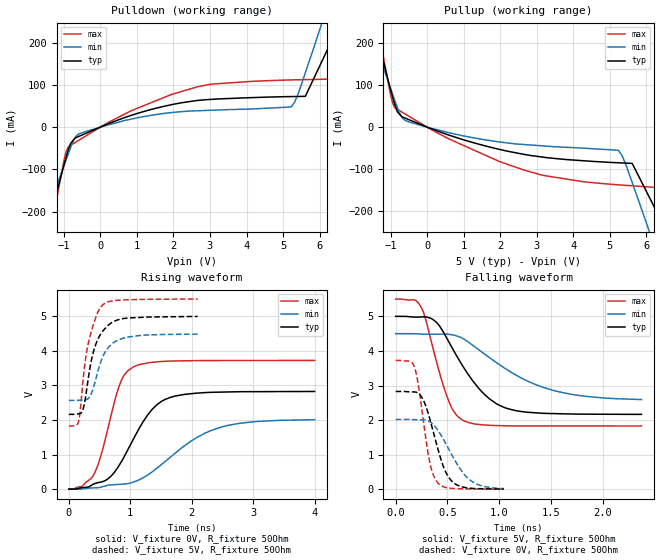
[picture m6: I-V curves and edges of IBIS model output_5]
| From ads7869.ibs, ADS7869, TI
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|   output_5 Model
[Model]   output_5
Model_type   Output
Polarity   Non-Inverting
Vmeas = 2.5
Vref = 2.5
Cref = 30pF
Rref = 50
|   typ   min   max
|   (nom PVT)   (fast PVT)   (slow PVT)
|C_comp from frequency sweep method (F=8MHz)
|C_comp   3.715e-12   3.568e-12   3.796e-12
|ON state : BUFFER OUTPUT TURNED HIGH
|C_comp   3.715e-12   3.568e-12   3.796e-12
|OFF state: BUFFER OUTPUT TURNED LOW
|C_comp   3.208e-12   3.054e-12   3.276e-12
|C_comp from LC tank measurement(L=1nH)
|Resonant Frequency(Hz)   3.030e+09   3.070e+09   2.990e+09
C_comp   2.762e-12   2.690e-12   2.836e-12
|ON state : BUFFER OUTPUT TURNED HIGH
|Resonant Frequency(Hz)   3.030e+09   3.070e+09   2.990e+09
|C_comp   2.762e-12   2.690e-12   2.836e-12
|OFF state: BUFFER OUTPUT TURNED LOW
|Resonant Frequency(Hz)   3.030e+09   3.080e+09   2.940e+09
|C_comp   2.762e-12   2.673e-12   2.933e-12
| Where nom  PVT is Nominal Process, 5V, 36C
|   Fast PVT is Strong Process,  5.5V, -40C
|   Slow PVT is Weak Process,   4.5V, 96C
[Voltage Range]   5   4.5   5.5
|Ambient Temperature   25   85   -40
|Junction Temperature
[Temperature Range]   36   96   -40
[Pullup Reference]   5   4.5   5.5
[Pulldown Reference]   0   0   0
[Power Clamp Reference]   5   4.5   5.5
[GND Clamp Reference]   0   0   0
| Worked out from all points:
|   slope of the pulldown table from 0 to 0.75 V, typ, clamps not added: 29.9 ohm
|   slope of the pullup table from 0 to 0.75 V, typ, clamps not added: 32.1 ohm
|   falling waveform, V_fixture 5V, R_fixture 50Ohm: 20-80 % time 380ps typ, 636ps min, 208ps max; typ from 5 V to 2.17 V
|   rising waveform, V_fixture 0V, R_fixture 50Ohm: 20-80 % time 562ps typ, 927ps min, 337ps max; typ from 0 V to 2.83 V
|   rising waveform, V_fixture 5V, R_fixture 50Ohm: 20-80 % time 221ps typ, 242ps min, 199ps max; typ from 2.16 V to 5 V
|   falling waveform, V_fixture 0V, R_fixture 50Ohm: 20-80 % time 165ps typ, 239ps min, 111ps max; typ from 2.83 V to 0.007 V
[Pulldown]
|   Voltage   I(typ)   I(min)   I(max)
-5V       -1.419A    -1.099A    -1.948A
-1.25V    -173.3mA   -154.1mA   -193.6mA
-930mV    -69.19mA   -75.45mA   -56.37mA
-815mV    -38.74mA   -48.41mA   -42.97mA
-536mV    -19.88mA   -14.34mA   -28.17mA
2.645V    63.01mA    38.7mA     95.13mA
5.22V     72.29mA    47.68mA    111.8mA
5.61V     72.9mA     128.4mA    112.4mA
6.034V    150.3mA    238.4mA    113.1mA
6.423V    248.9mA    340.7mA    115.4mA
6.66V     329.7mA    402.9mA    180.6mA
10V       1.472A     1.282A     1.753A
[Pullup]
|   Voltage   I(typ)   I(min)   I(max)
-5V       1.465A     1.147A     1.975A
-1.25V    172.6mA    155.4mA    189.1mA
-941mV    69.28mA    76.16mA    55.81mA
-671mV    23.77mA    20.75mA    34.67mA
-392mV    13.81mA    9.597mA    20.14mA
2.645V    -64.6mA    -41.24mA   -101.8mA
5.224V    -84.5mA    -54.85mA   -136.9mA
5.61V     -86.04mA   -131.4mA   -139.2mA
6.034V    -158.5mA   -236.2mA   -141.7mA
6.423V    -252.6mA   -333.6mA   -145.8mA
6.688V    -339.6mA   -399.8mA   -212.4mA
10V       -1.432A    -1.231A    -1.748A
[Ramp]
R_load = 50
|   typ   min   max
dV/dt_r   1.69569/5.61952e-10   1.20577/9.26732e-10   2.23404/3.37272e-10
dV/dt_f   1.70155/3.80038e-10   1.15899/6.51551e-10   2.20473/2.08222e-10
[Falling Waveform]
V_fixture = 5V
V_fixture_min = 4.5V
V_fixture_max = 5.5V
R_fixture = 50Ohm
|   Time   V(typ)   V(min)   V(max)
0s        5V         4.5V       5.5V
243.5ps   4.982V     4.488V     5.28V
372.4ps   4.881V     4.483V     3.935V
485.6ps   4.411V     4.487V     2.763V
561.5ps   4V         4.458V     2.246V
648.2ps   3.561V     4.36V      1.997V
858.2ps   2.741V     3.911V     1.858V
1.084ns   2.329V     3.442V     1.834V
1.604ns   2.182V     2.799V     1.83V
2.374ns   2.165V     2.593V     1.829V
[Rising Waveform]
V_fixture = 0V
V_fixture_min = 0V
V_fixture_max = 0V
R_fixture = 50Ohm
|   Time   V(typ)   V(min)   V(max)
0s        1.133nV    9.184nV    1.013nV
209.9ps   41.68mV    6.018mV    77.86mV
408.2ps   150.7mV    37.86mV    428.4mV
539.7ps   212.3mV    67.83mV    1.079V
807.7ps   656.3mV    137.6mV    2.922V
1.038ns   1.403V     196.1mV    3.523V
1.359ns   2.315V     504.1mV    3.669V
1.731ns   2.694V     1.041V     3.71V
2.534ns   2.81V      1.82V      3.721V
4ns       2.826V     2.01V      3.723V
[Rising Waveform]
V_fixture = 5V
V_fixture_min = 4.5V
V_fixture_max = 5.5V
R_fixture = 50Ohm
|   Time   V(typ)   V(min)   V(max)
0s        2.164V     2.568V     1.825V
159.1ps   2.178V     2.571V     1.958V
184.8ps   2.188V     2.575V     2.253V
234.3ps   2.325V     2.581V     3.19V
307.6ps   3.09V      2.612V     4.136V
404.9ps   4.001V     2.959V     4.789V
539.7ps   4.542V     3.775V     5.312V
692.9ps   4.812V     4.189V     5.441V
913.9ps   4.94V      4.38V      5.475V
2.097ns   4.997V     4.485V     5.499V
[Falling Waveform]
V_fixture = 0V
V_fixture_min = 0V
V_fixture_max = 0V
R_fixture = 50Ohm
|   Time   V(typ)   V(min)   V(max)
0s        2.826V     2.017V     3.723V
134.3ps   2.816V     2.018V     3.702V
184.8ps   2.812V     2.011V     3.502V
253.6ps   2.655V     2.007V     2.289V
323.8ps   2.093V     1.962V     853.2mV
408.2ps   1.16V      1.704V     178.3mV
475.5ps   546mV      1.367V     57.24mV
568.7ps   164.8mV    853.5mV    19.62mV
756ps     21.78mV    188mV      7.598mV
1.044ns   6.651mV    18.93mV    1.761mV
